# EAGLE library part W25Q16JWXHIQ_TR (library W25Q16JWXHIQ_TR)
SPIFLASH, 1.8V, 16M-BIT, 4KB UNIFORM SECTOR Source: Datasheet
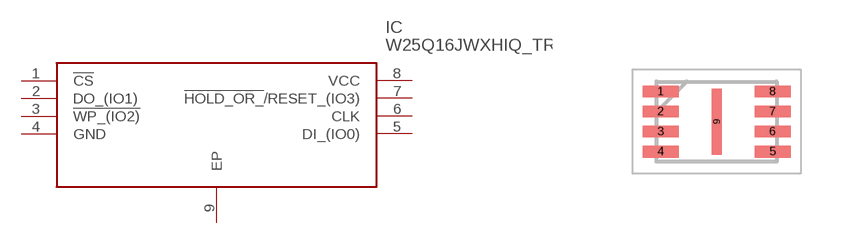
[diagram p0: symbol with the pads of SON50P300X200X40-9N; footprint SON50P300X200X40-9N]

Designator prefix IC

## W25Q16JWXHIQ_TR (Description: SPIFLASH, 1.8V, 16M-BIT, 4KB UNIFORM SECTOR; Height: 0.4mm; Manufacturer_Name: Winbond; Manufacturer_Part_Number: W25Q16JWXHIQ TR; Mouser_Part_Number: 454-W25Q16JWXHIQTR; Mouser_Price-Stock: https://www.mouser.co.uk/ProductDetail/Winbond/W25Q16JWXHIQ-TR?qs=YwPsRIUVAOdYBeCP6UUmNw%3D%3D)  [SON50P300X200X40-9N]
1  !CS
2  DO_(IO1)
3  !WP_(IO2)
4  GND
5  DI_(IO0)
6  CLK
7  !HOLD_OR_!/RESET_(IO3)
8  VCC
9  EP

## Footprint SON50P300X200X40-9N (pad centres in mm)
8-Pad XSON 2x3x0.4-mm
smd 0.9 x 0.3: 1 -1.4,0.75; 2 -1.4,0.25; 3 -1.4,-0.25; 4 -1.4,-0.75; 5 1.4,-0.75; 6 1.4,-0.25; 7 1.4,0.25; 8 1.4,0.75
smd 0.25 x 1.65: 9 0,0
